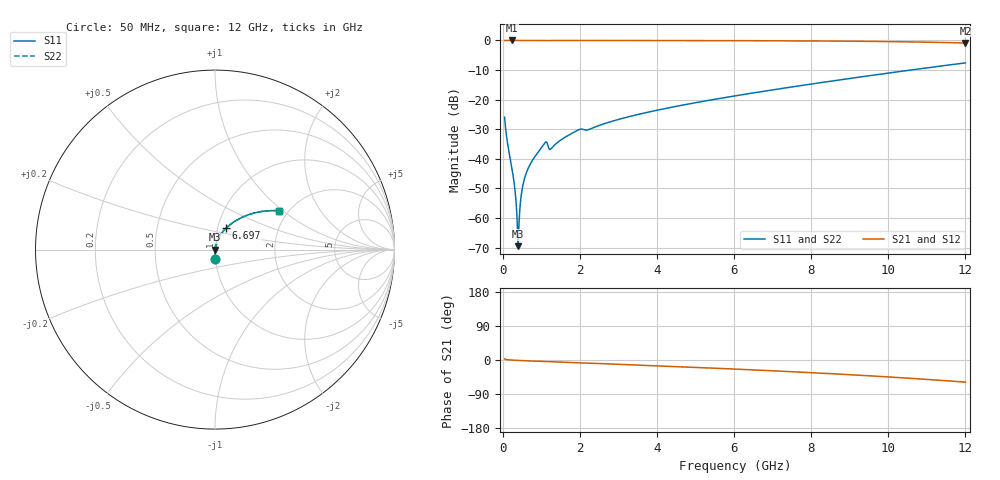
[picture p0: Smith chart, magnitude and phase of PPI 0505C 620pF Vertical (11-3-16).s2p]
# GHz S MA R 50
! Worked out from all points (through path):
!   1601 points, 50 MHz to 12 GHz, reference 50 ohm
!   highest |S21| = 0.00 dB at 236.7 MHz (marker M1); lowest = -0.9 dB at 12 GHz (marker M2)
!   group delay of S21, straight-line fit = 13.1 ps
!   lowest |S11| = -69.5 dB at 401 MHz (marker M3), VSWR 1.00, Z = 50 + j0.00168 ohm
!   |S11| at or under -10 dB: start of sweep to 10.58 GHz
!   |S22| runs from -69.5 to -7.6 dB; largest |S21 - S12| = 0
!   S11 on the Smith chart (normalised r, x): 50 MHz: 1.00, -0.10; 6.697 GHz: 1.10, +0.27; 12 GHz: 1.80, +0.94
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0.05  0.05042 -87.0  0.9985 2.7  0.9985 2.7  0.05042 -87.0
0.2367188  0.007067 -88.0  0.9997 -0.3  0.9997 -0.3  0.007067 -88.0
0.3039375  0.003601 -85.8  0.9997 -0.7  0.9997 -0.7  0.003601 -85.8
0.3636875  0.00128 -76.4  0.9997 -1.0  0.9997 -1.0  0.00128 -76.4
0.4010313  0.0003339 2.9  0.9996 -1.2  0.9996 -1.2  0.0003339 2.9
0.438375  0.001226 72.4  0.9996 -1.3  0.9996 -1.3  0.001226 72.4
0.498125  0.002882 81.2  0.9996 -1.6  0.9996 -1.6  0.002882 81.2
0.5728125  0.00479 83.5  0.9996 -1.9  0.9996 -1.9  0.00479 83.5
0.6848437  0.007438 84.3  0.9995 -2.4  0.9995 -2.4  0.007438 84.3
0.8491562  0.01121 84.1  0.9993 -3.1  0.9993 -3.1  0.01121 84.1
1.095625  0.01868 75.1  0.9963 -4.2  0.9963 -4.2  0.01868 75.1
1.252469  0.01469 73.5  0.9967 -4.5  0.9967 -4.5  0.01469 73.5
1.588563  0.02249 81.6  0.9987 -5.9  0.9987 -5.9  0.02249 81.6
2.044156  0.03183 74.3  0.995 -7.7  0.995 -7.7  0.03183 74.3
2.215937  0.03095 75.7  0.9961 -8.2  0.9961 -8.2  0.03095 75.7
2.962813  0.04549 77.5  0.9977 -11.2  0.9977 -11.2  0.04549 77.5
4.038312  0.06695 73.6  0.9965 -15.5  0.9965 -15.5  0.06695 73.6
6.025  0.1157 65.4  0.9917 -23.9  0.9917 -23.9  0.1157 65.4
6.697188  0.1361 62.4  0.9889 -27.0  0.9889 -27.0  0.1361 62.4
8.019156  0.184 56.0  0.9808 -33.5  0.9808 -33.5  0.184 56.0
10.01331  0.2816 44.8  0.9568 -44.7  0.9568 -44.7  0.2816 44.8
12  0.4177 31.2  0.9048 -58.4  0.9048 -58.4  0.4177 31.2
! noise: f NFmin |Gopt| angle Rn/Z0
0.05  0.0003025  0.8289  0.1962  0.0003722
1.372  0.00441  0.7007  3.914  0.002882
2.701  0.005711  0.5784  7.462  0.002452
4.031  0.006707  0.4945  10.64  0.002266
5.36  0.008282  0.4678  13.72  0.002597
6.682  0.01002  0.4584  16.63  0.003049
8.012  0.01198  0.4606  19.46  0.003644
9.341  0.01428  0.473  22.23  0.004445
10.67  0.01704  0.4948  25.03  0.005565
12  0.02052  0.5258  27.93  0.007203
